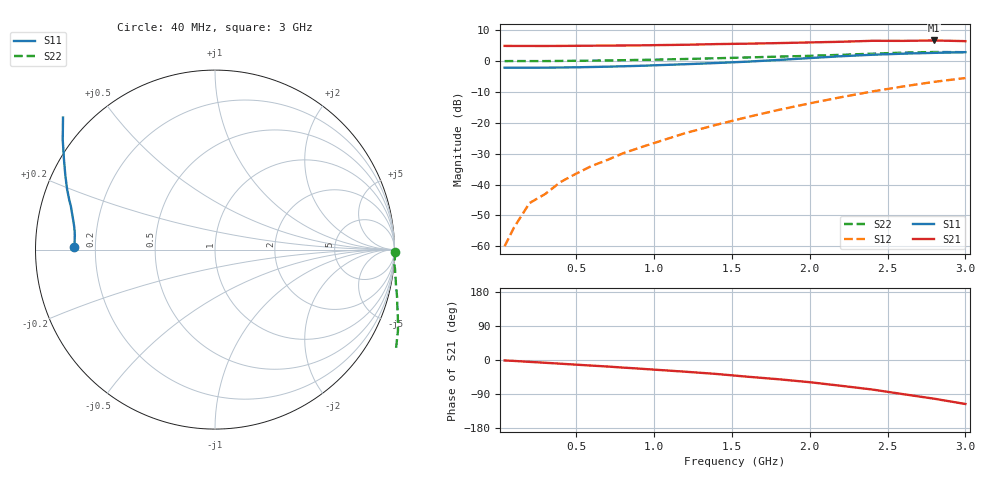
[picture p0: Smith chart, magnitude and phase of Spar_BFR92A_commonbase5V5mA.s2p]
! Filename:  BFR92ACB.S2P  Version:  2.0
! NXP part #: BFR92A  Date: Jul 1990
! Bias condition: Vce=5V, Ic=5mA
! COMMON BASE
#  MHz  S  MA  R  50
! Freq  S11  S21  S12  S22
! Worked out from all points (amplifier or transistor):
!   21 points, 40 MHz to 3 GHz, reference 50 ohm
!   highest |S21| = 6.7 dB at 2.8 GHz (marker M1)
!   |S21| within 3 dB of that: start of sweep to end of sweep
!   unconditionally stable (mu >= 1): nowhere
!   at 300 MHz: K = -0.44, MSG = 24.0 dB, |S12| = -43.1 dB
!   at 1 GHz: K = -0.91, MSG = 15.9 dB, |S12| = -26.6 dB
!   at 3 GHz: K = -0.77, MSG = 6.0 dB, |S12| = -5.5 dB
40  0.784 179.1  1.768 -1.2  0.001 61.9  1.002 -0.7
100  0.783 177.9  1.765 -2.4  0.002 84.5  1.004 -1.4
200  0.784 176.0  1.764 -4.9  0.005 104.4  1.003 -3.1
300  0.785 174.2  1.762 -7.3  0.007 113.2  1.003 -4.7
400  0.789 172.5  1.767 -9.8  0.011 122.2  1.009 -6.2
500  0.795 170.7  1.772 -12.3  0.015 125.1  1.014 -7.8
600  0.804 168.8  1.782 -14.8  0.02 129.6  1.02 -9.3
700  0.814 167.0  1.788 -17.2  0.025 132.6  1.027 -11.0
800  0.826 165.1  1.795 -20.0  0.032 134.8  1.036 -12.6
900  0.839 163.2  1.802 -22.6  0.039 137.4  1.047 -14.4
1000  0.856 161.4  1.818 -25.4  0.047 139.0  1.057 -16.2
1200  0.892 157.6  1.844 -30.9  0.068 141.0  1.084 -20.0
1400  0.933 153.4  1.891 -36.8  0.093 140.7  1.115 -23.9
1600  0.982 149.0  1.921 -44.1  0.124 140.4  1.148 -28.5
1800  1.046 144.2  1.963 -50.8  0.162 138.4  1.185 -33.7
2000  1.122 139.0  2.012 -58.6  0.207 135.6  1.22 -39.9
2200  1.201 133.8  2.062 -68.0  0.26 132.1  1.266 -47.2
2400  1.27 127.8  2.138 -77.8  0.322 127.1  1.322 -55.3
2600  1.323 120.3  2.132 -90.1  0.389 121.7  1.374 -64.0
2800  1.364 111.0  2.166 -102.2  0.462 114.7  1.407 -72.9
3000  1.4 101.3  2.111 -116.1  0.533 107.7  1.399 -82.6
